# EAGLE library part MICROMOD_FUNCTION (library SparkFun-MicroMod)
MicroMod Connector Description: A card edge connector and mating PCB connector to allow various MicroMod Processor Boards to be coupled with various carrier boards of different capabilities. Based on the M.2 standard.
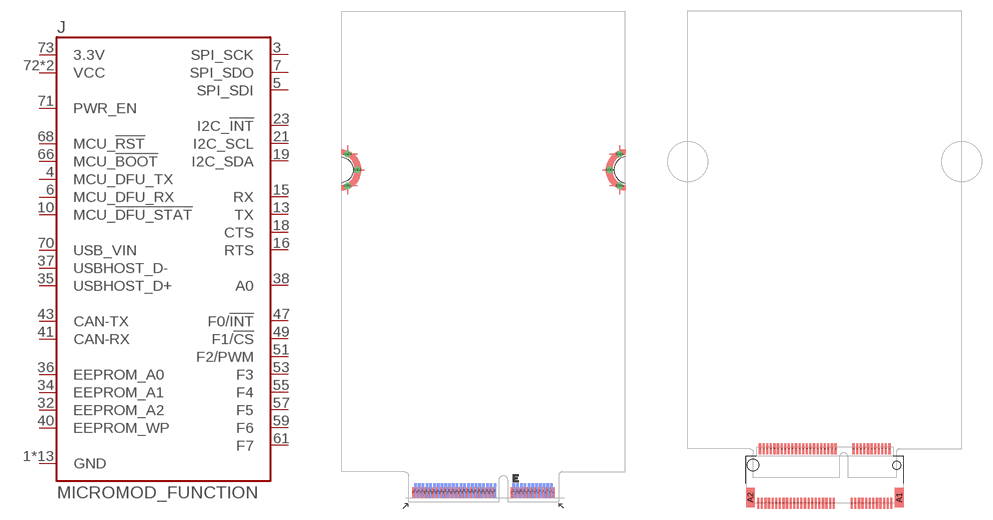
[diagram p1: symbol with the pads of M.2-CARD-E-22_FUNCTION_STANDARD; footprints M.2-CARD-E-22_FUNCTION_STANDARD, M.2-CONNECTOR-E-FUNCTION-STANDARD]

Designator prefix J

## MICROMOD_FUNCTION_STANDARD  [M.2-CARD-E-22_FUNCTION_STANDARD]
1  GND
2  GND
3  SPI_SCK
4  MCU_DFU_TX
5  SPI_SDI
6  MCU_DFU_RX
7  SPI_SDO
8  GND
10  MCU_!DFU_STAT!
13  TX
15  RX
16  RTS
18  CTS
19  I2C_SDA
21  I2C_SCL
23  I2C_!INT!
32  EEPROM_A2
33  GND
34  EEPROM_A1
35  USBHOST_D+
36  EEPROM_A0
37  USBHOST_D-
38  A0
39  GND
40  EEPROM_WP
41  CAN-RX
43  CAN-TX
45  GND
47  F0/!INT!
49  F1/!CS!
51  F2/PWM
53  F3
55  F4
57  F5
59  F6
61  F7
66  MCU_!BOOT!
68  MCU_!RST!
70  USB_VIN
71  PWR_EN
72  VCC
73  3.3V
74  VCC
75  GND
GND1  GND
GND2  GND
GND3  GND
GND4  GND
GND5  GND
GND6  GND

## MICROMOD_FUNCTION_MAIN (PROD_ID: CONN-14877)  [M.2-CONNECTOR-E-FUNCTION-STANDARD]
1  GND
2  GND
3  SPI_SCK
4  MCU_DFU_TX
5  SPI_SDI
6  MCU_DFU_RX
7  SPI_SDO
8  GND
10  MCU_!DFU_STAT!
13  TX
15  RX
16  RTS
18  CTS
19  I2C_SDA
21  I2C_SCL
23  I2C_!INT!
32  EEPROM_A2
33  GND
34  EEPROM_A1
35  USBHOST_D+
36  EEPROM_A0
37  USBHOST_D-
38  A0
39  GND
40  EEPROM_WP
41  CAN-RX
43  CAN-TX
45  GND
47  F0/!INT!
49  F1/!CS!
51  F2/PWM
53  F3
55  F4
57  F5
59  F6
61  F7
66  MCU_!BOOT!
68  MCU_!RST!
70  USB_VIN
71  PWR_EN
72  VCC
73  3.3V
74  VCC
75  GND

## Footprint M.2-CARD-E-22_FUNCTION_STANDARD (pad centres in mm)
smd 0.35 x 1.45: 1 9.25,1.275; 3 8.75,1.275; 5 8.25,1.275; 7 7.75,1.275; 9 7.25,1.275; 11 6.75,1.275; 13 6.25,1.275; 15 5.75,1.275; 17 5.25,1.275; 19 4.75,1.275; 21 4.25,1.275; 23 3.75,1.275; 33 1.25,1.275; 35 0.75,1.275; 37 0.25,1.275; 39 -0.25,1.275; 41 -0.75,1.275; 43 -1.25,1.275; 45 -1.75,1.275; 47 -2.25,1.275; 49 -2.75,1.275; 51 -3.25,1.275; 53 -3.75,1.275; 55 -4.25,1.275; 57 -4.75,1.275; 59 -5.25,1.275; 61 -5.75,1.275; 63 -6.25,1.275; 65 -6.75,1.275; 67 -7.25,1.275; 69 -7.75,1.275; 71 -8.25,1.275; 73 -8.75,1.275; 75 -9.25,1.275
smd 0.35 x 1.95 bottom: 2 9,1.525; 4 8.5,1.525; 6 8,1.525; 8 7.5,1.525; 10 7,1.525; 12 6.5,1.525; 14 6,1.525; 16 5.5,1.525; 18 5,1.525; 20 4.5,1.525; 22 4,1.525; 32 1.5,1.525; 34 1,1.525; 36 0.5,1.525; 38 0,1.525; 40 -0.5,1.525; 42 -1,1.525; 44 -1.5,1.525; 46 -2,1.525; 48 -2.5,1.525; 50 -3,1.525; 52 -3.5,1.525; 54 -4,1.525; 56 -4.5,1.525; 58 -5,1.525; 60 -5.5,1.525; 62 -6,1.525; 64 -6.5,1.525; 66 -7,1.525; 68 -7.5,1.525; 70 -8,1.525; 72 -8.5,1.525; 74 -9,1.525
drill 0.305 pad 0.61: GND1 -18,41.9; GND2 -16.7,44; GND3 -18,46.1; GND4 18,41.9; GND5 16.7,44; GND6 18,46.1

## Footprint M.2-CONNECTOR-E-FUNCTION-STANDARD (pad centres in mm)
smd 0.3 x 1.55: 1 9.25,-5.275; 2 9,2.275; 3 8.75,-5.275; 4 8.5,2.275; 5 8.25,-5.275; 6 8,2.275; 7 7.75,-5.275; 8 7.5,2.275; 9 7.25,-5.275; 10 7,2.275; 11 6.75,-5.275; 12 6.5,2.275; 13 6.25,-5.275; 14 6,2.275; 15 5.75,-5.275; 16 5.5,2.275; 17 5.25,-5.275; 18 5,2.275; 19 4.75,-5.275; 20 4.5,2.275; 21 4.25,-5.275; 22 4,2.275; 23 3.75,-5.275; 32 1.5,2.275; 33 1.25,-5.275; 34 1,2.275; 35 0.75,-5.275; 36 0.5,2.275; 37 0.25,-5.275; 38 0,2.275; 39 -0.25,-5.275; 40 -0.5,2.275; 41 -0.75,-5.275; 42 -1,2.275; 43 -1.25,-5.275; 44 -1.5,2.275; 45 -1.75,-5.275; 46 -2,2.275; 47 -2.25,-5.275; 48 -2.5,2.275; 49 -2.75,-5.275; 50 -3,2.275; 51 -3.25,-5.275; 52 -3.5,2.275; 53 -3.75,-5.275; 54 -4,2.275; 55 -4.25,-5.275; 56 -4.5,2.275; 57 -4.75,-5.275; 58 -5,2.275; 59 -5.25,-5.275; 60 -5.5,2.275; 61 -5.75,-5.275; 62 -6,2.275; 63 -6.25,-5.275; 64 -6.5,2.275; 65 -6.75,-5.275; 66 -7,2.275; 67 -7.25,-5.275; 68 -7.5,2.275; 69 -7.75,-5.275; 70 -8,2.275; 71 -8.25,-5.275; 72 -8.5,2.275; 73 -8.75,-5.275; 74 -9,2.275; 75 -9.25,-5.275
smd 1.2 x 2.75: A1 10.35,-4.5; A2 -10.35,-4.5
hole 1.1 at 10,0
hole 1.6 at -10,0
